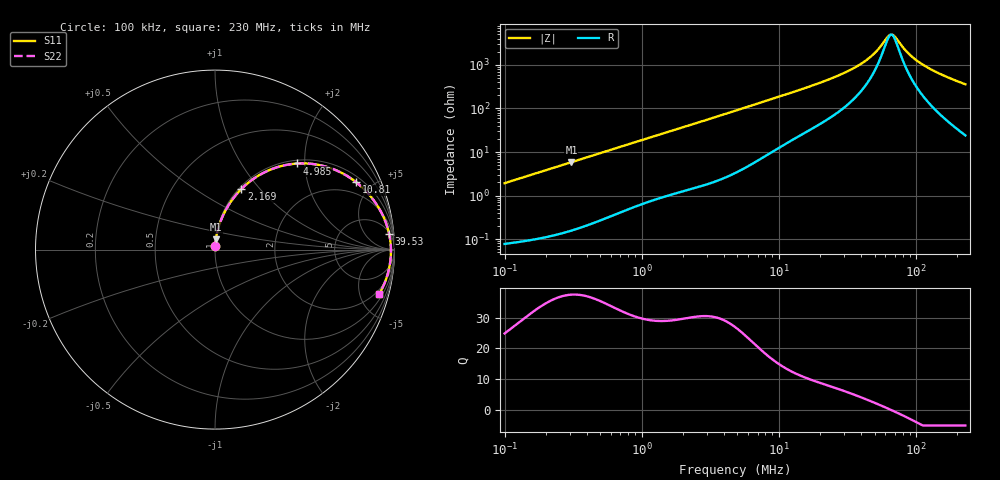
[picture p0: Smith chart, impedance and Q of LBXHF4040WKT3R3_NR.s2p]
! LBXHF4040WKT3R3_NR  S-PARAMETER MODEL  ( Standard Model )
! Model Generated by TAIYO YUDEN Corporation (http://www.ty-top.com)
! Version 1.0
! TAIYO YUDEN Control No. 20221109
! Copyright(c) 2022 TAIYO YUDEN CO.,LTD. All Rights Reserved.
! Product Description (link to TY-COMPAS)
! https://ds.yuden.co.jp/TYCOMPAS/or/detail?pn=LBXHF4040WKT3R3MNR&u=M
! Products Name : Inductors
! Characteristics :
!  Inductance : 3.3 [uH] , SRF(min) : 45 [MHz] , DC Resistance(max) : 0.066 [Ohm]
!  Rated Current : Saturation  2400 [mA] , Temp Rise  1700 [mA]
!  Case Size : 4.0 x 4.0 / 0.157 x 0.157 [mm/inch] , Thickness : 2.0 / 0.079 [mm/inch]
!  (Conditions: Temperature = 25 [degC] , DC Bias Current = 0 [A])
! External Node Assignments :
!  1  o---GGG---o  2
! GND o---------o GND
! Frequency Range : 0.1MHz  -  229.966873MHz  [ 402 STEP ]
# MHz S RI R 50
! Freq[MHz].  S11 Real  S11 Imag  S21 Real  S21 Imag  S12 Real  S12 Imag  S22 Real  S22 Imag
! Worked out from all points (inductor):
!   401 points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, 100 kHz to 230 MHz, reference 50 ohm
!   read as one part in series: L = 3.06 uH near 103.9 kHz
!   highest Q = 37.4 at 307.2 kHz (marker M1), where L = 3.04 uH
!   self-resonance near 66.22 MHz
!   S11 on the Smith chart (normalised r, x): 100 kHz: 1.00, +0.04; 2.169 MHz: 1.03, +0.80; 4.985 MHz: 1.07, +1.83; 10.81 MHz: 1.29, +4.02; 39.53 MHz: 6, +20; 230 MHz: 1.48, -7.16
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0.1  0.00115 0.0192  0.9989 -0.0192  0.9989 -0.0192  0.00115 0.0192
0.307214  0.00498 0.0583  0.995 -0.0583  0.995 -0.0583  0.00498 0.0583
0.365661  0.00668 0.0691  0.9933 -0.0691  0.9933 -0.0691  0.00668 0.0691
0.719821  0.0222 0.1324  0.9778 -0.1324  0.9778 -0.1324  0.0222 0.1324
1.337081  0.0655 0.2307  0.9345 -0.2307  0.9345 -0.2307  0.0655 0.2307
2.169012  0.1462 0.3369  0.8538 -0.3369  0.8538 -0.3369  0.1462 0.3369
3.194076  0.2632 0.4242  0.7368 -0.4242  0.7368 -0.4242  0.2632 0.4242
4.889189  0.4495 0.479  0.5505 -0.479  0.5505 -0.479  0.4495 0.479
4.984722  0.4589 0.4797  0.5411 -0.4797  0.5411 -0.4797  0.4589 0.4797
7.061808  0.6246 0.4603  0.3754 -0.4603  0.3754 -0.4603  0.6246 0.4603
10.80955  0.786 0.3759  0.214 -0.3759  0.214 -0.3759  0.786 0.3759
17.53523  0.8961 0.2578  0.1039 -0.2578  0.1039 -0.2578  0.8961 0.2578
27.90047  0.9501 0.1552  0.0499 -0.1552  0.0499 -0.1552  0.9501 0.1552
39.52632  0.9701 0.0885  0.0299 -0.0885  0.0299 -0.0885  0.9701 0.0885
49.85818  0.9771 0.0478  0.0229 -0.0478  0.0229 -0.0478  0.9771 0.0478
64.11956  0.9803 0.0054  0.0197 -0.0054  0.0197 -0.0054  0.9803 0.0054
66.6498  0.9804 -0.00107  0.0196 0.00107  0.0196 0.00107  0.9804 -0.00107
69.27989  0.9805 -0.00755  0.0195 0.00755  0.0195 0.00755  0.9805 -0.00755
89.09663  0.9784 -0.0504  0.0216 0.0504  0.0216 0.0504  0.9784 -0.0504
112.3857  0.9726 -0.0922  0.0274 0.0922  0.0274 0.0922  0.9726 -0.0922
156.1644  0.9553 -0.1582  0.0447 0.1582  0.0447 0.1582  0.9553 -0.1582
229.9669  0.9136 -0.2493  0.0864 0.2493  0.0864 0.2493  0.9136 -0.2493
